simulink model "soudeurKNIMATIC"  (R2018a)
settings: Solver=VariableStepAuto  StartTime=0.0  StopTime=inf  RelTol=1e-3
StartFcn:
  | myStartFcn
model workspace: external: MATLAB File (data not in the file)
undefined symbols (not defined in the file or in its folder): deg, kg, m, mm, N, rad, s, sigbuilder_block, smiData, X, Y, Z
libraries: sm_lib x59, nesl_utility x13, robotcorelib x1, robotmaniplib x1
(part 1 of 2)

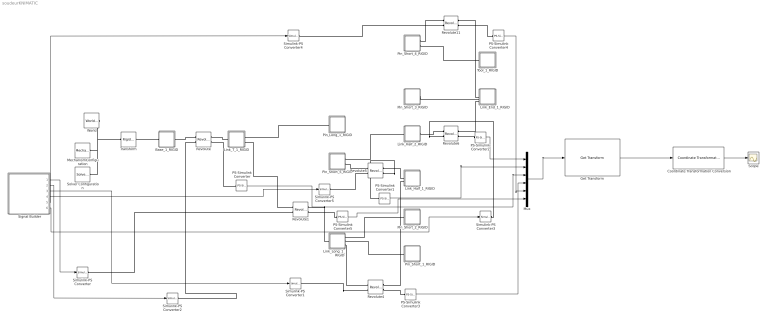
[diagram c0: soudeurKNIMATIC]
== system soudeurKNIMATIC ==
  Base_1_RIGID : Subsystem
  Coordinate Transformation Conversion : robotcorelib/Coordinate Transformation Conversion  InputRepresentation=Quaternion  InputEulerSequence=ZYX  ShowTrVecInputPort=on  OutputRepresentation=Rotation Matrix  OutputEulerSequence=ZYX  ShowTrVecOutputPort=on  SimulateUsing=Interpreted execution
  Get Transform : robotmaniplib/Get Transform  RigidBodyTree=twoJointRigidBodyTree  SourceBody=base  TargetBody=base
  Link_End_1_RIGID : Subsystem
  Link_Half_1_RIGID : Subsystem
  Link_Half_2_RIGID : Subsystem
  Link_Long_1_RIGID : Subsystem
  Link_T_1_RIGID : Subsystem
  MechanismConfiguration : sm_lib/Utilities/Mechanism Configuration  UniformGravity=Constant  GravityVector=[0 -9.80665 0]  GravityUnits=m/s^2  LinearizationDelta=0.001
  Mux : Mux  Inputs=6
  PS-Simulink Converter{,1..5} (6 alike) : nesl_utility/PS-Simulink Converter  PhysicalDomain=network_engine_domain  SubClassName=ps_output  LeftPortType=input  RightPortType=output  PseudoPeriodic=off  Frequencies=[]  Unit=1  AffineConversion=off
  Pin_Long_1_RIGID : Subsystem
  Pin_Short_1_RIGID : Subsystem
  Pin_Short_2_RIGID : Subsystem
  Pin_Short_3_RIGID : Subsystem
  Pin_Short_4_RIGID : Subsystem
  Pin_Short_5_RIGID : Subsystem
  Revolute : sm_lib/Joints/Revolute Joint  SenseConstraintForce=off  SenseConstraintForceX=off  SenseConstraintForceY=off  SenseConstraintForceZ=off  SenseConstraintTorque=off  SenseConstraintTorqueX=off  SenseConstraintTorqueY=off  SenseConstraintTorqueZ=off  SenseTotalForce=off  SenseTotalForceX=off  SenseTotalForceY=off  SenseTotalForceZ=off  SenseTotalTorque=off  SenseTotalTorqueX=off  SenseTotalTorqueY=off  SenseTotalTorqueZ=off  CompositeWrenchDir=FollowerOnBase  CompositeWrenchFrame=BaseFrame  EquilibriumPosition=0  EquilibriumPositionUnits=rad  SpringStiffness=0  SpringStiffnessUnits=N*m/rad  DampingCoefficient=0  DampingCoefficientUnits=N*m/(rad/s)  TorqueActuationMode=ComputedTorque  MotionActuationMode=InputMotion  SensePosition=on  SenseVelocity=off  SenseAcceleration=off  SenseTorqueForce=off  PositionTargetSpecify=on  PositionTargetPriority=Low  PositionTargetValue=smiData.RevoluteJoint(1).Rz.Pos  PositionTargetValueUnits=deg  VelocityTargetSpecify=off  VelocityTargetPriority=High  VelocityTargetValue=0  VelocityTargetValueUnits=deg/s
  Revolute1 : sm_lib/Joints/Revolute Joint  SenseConstraintForce=off  SenseConstraintForceX=off  SenseConstraintForceY=off  SenseConstraintForceZ=off  SenseConstraintTorque=off  SenseConstraintTorqueX=off  SenseConstraintTorqueY=off  SenseConstraintTorqueZ=off  SenseTotalForce=off  SenseTotalForceX=off  SenseTotalForceY=off  SenseTotalForceZ=off  SenseTotalTorque=off  SenseTotalTorqueX=off  SenseTotalTorqueY=off  SenseTotalTorqueZ=off  CompositeWrenchDir=FollowerOnBase  CompositeWrenchFrame=BaseFrame  EquilibriumPosition=0  EquilibriumPositionUnits=rad  SpringStiffness=0  SpringStiffnessUnits=N*m/rad  DampingCoefficient=0  DampingCoefficientUnits=N*m/(rad/s)  TorqueActuationMode=ComputedTorque  MotionActuationMode=InputMotion  SensePosition=on  SenseVelocity=off  SenseAcceleration=off  SenseTorqueForce=off  PositionTargetSpecify=on  PositionTargetPriority=Low  PositionTargetValue=smiData.RevoluteJoint(2).Rz.Pos  PositionTargetValueUnits=deg  VelocityTargetSpecify=off  VelocityTargetPriority=High  VelocityTargetValue=0  VelocityTargetValueUnits=deg/s
  Revolute11 : sm_lib/Joints/Revolute Joint  SenseConstraintForce=off  SenseConstraintForceX=off  SenseConstraintForceY=off  SenseConstraintForceZ=off  SenseConstraintTorque=off  SenseConstraintTorqueX=off  SenseConstraintTorqueY=off  SenseConstraintTorqueZ=off  SenseTotalForce=off  SenseTotalForceX=off  SenseTotalForceY=off  SenseTotalForceZ=off  SenseTotalTorque=off  SenseTotalTorqueX=off  SenseTotalTorqueY=off  SenseTotalTorqueZ=off  CompositeWrenchDir=FollowerOnBase  CompositeWrenchFrame=BaseFrame  EquilibriumPosition=0  EquilibriumPositionUnits=rad  SpringStiffness=0  SpringStiffnessUnits=N*m/rad  DampingCoefficient=0  DampingCoefficientUnits=N*m/(rad/s)  TorqueActuationMode=ComputedTorque  MotionActuationMode=InputMotion  SensePosition=on  SenseVelocity=off  SenseAcceleration=off  SenseTorqueForce=off  PositionTargetSpecify=on  PositionTargetPriority=Low  PositionTargetValue=smiData.RevoluteJoint(12).Rz.Pos  PositionTargetValueUnits=deg  VelocityTargetSpecify=off  VelocityTargetPriority=High  VelocityTargetValue=0  VelocityTargetValueUnits=deg/s
  Revolute4 : sm_lib/Joints/Revolute Joint  SenseConstraintForce=off  SenseConstraintForceX=off  SenseConstraintForceY=off  SenseConstraintForceZ=off  SenseConstraintTorque=off  SenseConstraintTorqueX=off  SenseConstraintTorqueY=off  SenseConstraintTorqueZ=off  SenseTotalForce=off  SenseTotalForceX=off  SenseTotalForceY=off  SenseTotalForceZ=off  SenseTotalTorque=off  SenseTotalTorqueX=off  SenseTotalTorqueY=off  SenseTotalTorqueZ=off  CompositeWrenchDir=FollowerOnBase  CompositeWrenchFrame=BaseFrame  EquilibriumPosition=0  EquilibriumPositionUnits=rad  SpringStiffness=0  SpringStiffnessUnits=N*m/rad  DampingCoefficient=0  DampingCoefficientUnits=N*m/(rad/s)  TorqueActuationMode=ComputedTorque  MotionActuationMode=InputMotion  SensePosition=on  SenseVelocity=off  SenseAcceleration=off  SenseTorqueForce=off  PositionTargetSpecify=on  PositionTargetPriority=Low  PositionTargetValue=smiData.RevoluteJoint(5).Rz.Pos  PositionTargetValueUnits=deg  VelocityTargetSpecify=off  VelocityTargetPriority=High  VelocityTargetValue=0  VelocityTargetValueUnits=deg/s
  Revolute5 : sm_lib/Joints/Revolute Joint  SenseConstraintForce=off  SenseConstraintForceX=off  SenseConstraintForceY=off  SenseConstraintForceZ=off  SenseConstraintTorque=off  SenseConstraintTorqueX=off  SenseConstraintTorqueY=off  SenseConstraintTorqueZ=off  SenseTotalForce=off  SenseTotalForceX=off  SenseTotalForceY=off  SenseTotalForceZ=off  SenseTotalTorque=off  SenseTotalTorqueX=off  SenseTotalTorqueY=off  SenseTotalTorqueZ=off  CompositeWrenchDir=FollowerOnBase  CompositeWrenchFrame=BaseFrame  EquilibriumPosition=0  EquilibriumPositionUnits=rad  SpringStiffness=0  SpringStiffnessUnits=N*m/rad  DampingCoefficient=0  DampingCoefficientUnits=N*m/(rad/s)  TorqueActuationMode=ComputedTorque  MotionActuationMode=InputMotion  SensePosition=on  SenseVelocity=off  SenseAcceleration=off  SenseTorqueForce=off  PositionTargetSpecify=on  PositionTargetPriority=Low  PositionTargetValue=smiData.RevoluteJoint(6).Rz.Pos  PositionTargetValueUnits=deg  VelocityTargetSpecify=off  VelocityTargetPriority=High  VelocityTargetValue=0  VelocityTargetValueUnits=deg/s
  Revolute6 : sm_lib/Joints/Revolute Joint  SenseConstraintForce=off  SenseConstraintForceX=off  SenseConstraintForceY=off  SenseConstraintForceZ=off  SenseConstraintTorque=off  SenseConstraintTorqueX=off  SenseConstraintTorqueY=off  SenseConstraintTorqueZ=off  SenseTotalForce=off  SenseTotalForceX=off  SenseTotalForceY=off  SenseTotalForceZ=off  SenseTotalTorque=off  SenseTotalTorqueX=off  SenseTotalTorqueY=off  SenseTotalTorqueZ=off  CompositeWrenchDir=FollowerOnBase  CompositeWrenchFrame=BaseFrame  EquilibriumPosition=0  EquilibriumPositionUnits=rad  SpringStiffness=0  SpringStiffnessUnits=N*m/rad  DampingCoefficient=0  DampingCoefficientUnits=N*m/(rad/s)  TorqueActuationMode=ComputedTorque  MotionActuationMode=InputMotion  SensePosition=on  SenseVelocity=off  SenseAcceleration=off  SenseTorqueForce=off  PositionTargetSpecify=on  PositionTargetPriority=Low  PositionTargetValue=smiData.RevoluteJoint(7).Rz.Pos  PositionTargetValueUnits=deg  VelocityTargetSpecify=off  VelocityTargetPriority=High  VelocityTargetValue=0  VelocityTargetValueUnits=deg/s
  Scope : Scope
  Signal Builder : Subsystem  Tag=STV Subsys  LoadFcn=sigbuilder_block('load');  StartFcn=sigbuilder_block('start');  StopFcn=sigbuilder_block('stop');  ClipboardFcn=sigbuilder_block('clipboard');  mask(Sigbuilder block){tuvar=[0:10]}
      mask help: Simulink:masks:SigbuilderBlock_MD
      mask init:
      | if ~strcmp(get_param(bdroot(gcbh),'SimulationStatus'),'stopped') tuvar = sigbuilder_block('maskInit'); end
  Simulink-PS Converter{,1..4} (5 alike) : nesl_utility/Simulink-PS Converter  PhysicalDomain=network_engine_domain  SubClassName=ps_input  LeftPortType=input  RightPortType=output  PseudoPeriodic=off  Frequencies=[]  NoiseDistribution=none  NoiseParameters=[]  Unit=rad  AffineConversion=off  FilteringAndDerivatives=filter  SimscapeFilterOrder=2  InputFilterTimeConstant=0.001  UdotUserProvided=0
  Simulink-PS Converter5 : nesl_utility/Simulink-PS Converter  PhysicalDomain=network_engine_domain  SubClassName=ps_input  LeftPortType=input  RightPortType=output  PseudoPeriodic=off  Frequencies=[]  NoiseDistribution=none  NoiseParameters=[]  Unit=1  AffineConversion=off  FilteringAndDerivatives=provide  SimscapeFilterOrder=1  InputFilterTimeConstant=0.001  UdotUserProvided=0
  Solver Configuration : nesl_utility/Solver Configuration  PhysicalDomain=network_engine_domain  SubClassName=solver  LeftPortType=input  RightPortType=generic  Tones=[]  Harmonics=[]  SimulateNoise=off  Profile=off  UseLocalSampling=off  EnableSwitchedLinearOptims=on  FrequencyDomain=off  UseCCode=off  RelTol=0.001  AbsTol=1e-06  MinStep=1e-09  ToWorkspace=off  RevertToSquareIcSolve=off  NumHomotopyIterations=100  PhasorMode=off  PhasorModeNumHarmonics=1  DoDC=off  ResidualTolerance=1e-09  UseLocalSolver=off  LocalSolverChoice=NE_BACKWARD_EULER_ADVANCER  LocalSolverSampleTime=0.001  DoFixedCost=off  MaxNonlinIter=3  MaxModeIter=2  LinearAlgebra=Sparse  EquationFormulation=NE_TIME_EF  DelaysMemoryBudget=1024  AutomaticFiltering=on  FilteringTimeConstant=0.001
  Tool_1_RIGID : Subsystem
  Transform : sm_lib/Frames and Transforms/Rigid Transform  TranslationMethod=Cartesian  TranslationStandardOffset=0  TranslationLengthUnit=mm  TranslationStandardAxis=+Z  TranslationCartesianOffset=smiData.RigidTransform(25).translation  TranslationROffset=0  TranslationROffsetUnits=m  TranslationZOffset=0  TranslationZOffsetUnits=m  TranslationThetaOffset=0  TranslationThetaOffsetUnits=deg  RotationMethod=ArbitraryAxis  RotationAngleUnits=rad  RotationStandardAxis=+Z  RotationAngle=smiData.RigidTransform(25).angle  RotationArbitraryAxis=smiData.RigidTransform(25).axis  FollAlignAxisA=+X  BaseAlignAxisA=+Y  FollAlignAxisB=+Y  BaseAlignAxisB=+Z  RotationSequenceAxes=FollowerAxes  RotationSequence=XYX  RotationSequenceAngles=[0 0 0]  RotationSequenceAnglesUnits=deg  RotationMatrix=[1 0 0; 0 1 0; 0 0 1]
  World : sm_lib/Frames and Transforms/World Frame
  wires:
  Signal Builder/1(Signal 1) -> Simulink-PS Converter/1
  Signal Builder/2(Signal 2) -> Simulink-PS Converter2/1
  Signal Builder/3(Signal 3) -> Simulink-PS Converter1/1
  Signal Builder/4(Signal 4) -> Simulink-PS Converter5/1
  Signal Builder/5(Signal 5) -> Simulink-PS Converter4/1
  Signal Builder/6(Signal 6) -> Simulink-PS Converter3/1
  Get Transform/1 -> Coordinate Transformation Conversion/1
  PS-Simulink Converter2/1 -> Mux/1
  PS-Simulink Converter1/1 -> Mux/2
  PS-Simulink Converter/1 -> Mux/3
  PS-Simulink Converter3/1 -> Mux/4
  PS-Simulink Converter4/1 -> Mux/5
  PS-Simulink Converter5/1 -> Mux/6
  Mux/1 -> Get Transform/1
  Coordinate Transformation Conversion/1 -> Scope/1
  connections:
  MechanismConfiguration/RConn1 -- Transform/LConn1 -- World/RConn1 -- Solver Configuration/RConn1
  Base_1_RIGID/RConn1 -- Revolute/LConn1
  Link_Half_1_RIGID/LConn2 -- Revolute4/RConn1
  Pin_Short_5_RIGID/RConn2 -- Revolute5/LConn1
  Link_Half_1_RIGID/LConn1 -- Revolute5/RConn1
  Link_Half_2_RIGID/RConn1 -- Revolute6/LConn1
  Link_End_1_RIGID/LConn3 -- Revolute6/RConn1
  Pin_Short_5_RIGID/RConn1 -- Link_Half_2_RIGID/LConn1
  Link_Long_1_RIGID/RConn2 -- Pin_Short_1_RIGID/LConn1
  Link_T_1_RIGID/LConn1 -- Revolute/RConn1
  Link_Long_1_RIGID/RConn1 -- Pin_Short_2_RIGID/LConn1
  Pin_Short_3_RIGID/RConn1 -- Link_End_1_RIGID/LConn2
  Pin_Short_4_RIGID/RConn1 -- Revolute11/LConn1
  Link_End_1_RIGID/LConn1 -- Revolute11/RConn1
  Base_1_RIGID/LConn1 -- Transform/RConn1
  Link_T_1_RIGID/RConn2 -- Revolute1/LConn1
  Link_Long_1_RIGID/LConn1 -- Revolute1/RConn1
  Link_T_1_RIGID/RConn1 -- Pin_Long_1_RIGID/LConn1
  Pin_Short_4_RIGID/RConn2 -- Tool_1_RIGID/LConn1
  Link_Long_1_RIGID/RConn3 -- Revolute4/LConn1
  Simulink-PS Converter/RConn1 -- Revolute1/LConn2
  Simulink-PS Converter2/RConn1 -- Revolute/LConn2
  Simulink-PS Converter5/RConn1 -- Revolute5/LConn2
  Simulink-PS Converter1/RConn1 -- Revolute4/LConn2
  Simulink-PS Converter3/RConn1 -- Revolute6/LConn2
  Simulink-PS Converter4/RConn1 -- Revolute11/LConn2
  PS-Simulink Converter/LConn1 -- Revolute/RConn2
  PS-Simulink Converter1/LConn1 -- Revolute5/RConn2
  PS-Simulink Converter2/LConn1 -- Revolute6/RConn2
  PS-Simulink Converter3/LConn1 -- Revolute4/RConn2
  PS-Simulink Converter4/LConn1 -- Revolute11/RConn2
  PS-Simulink Converter5/LConn1 -- Revolute1/RConn2

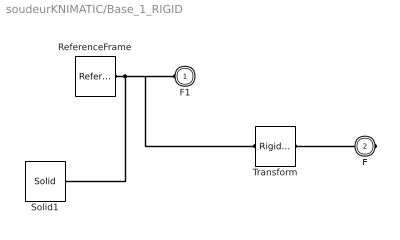
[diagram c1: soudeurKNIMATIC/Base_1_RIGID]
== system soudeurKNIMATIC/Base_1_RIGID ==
  ReferenceFrame : sm_lib/Frames and Transforms/Reference Frame
  Solid1 : sm_lib/Body Elements/Solid  InertiaType=Custom  Mass=smiData.Solid(4).mass  MassUnits=kg  CenterOfMass=smiData.Solid(4).CoM  CenterOfMassUnits=mm  MomentsOfInertia=smiData.Solid(4).MoI  MomentsOfInertiaUnits=kg*mm^2  ProductsOfInertia=smiData.Solid(4).PoI  ProductsOfInertiaUnits=kg*mm^2  DensityBased=on  Density=1000  DensityUnits=kg/m^3  DoExposeReferenceFrame=on  SerializedFrames=<Frames/>  GraphicType=FromGeometry  MarkerShape=Sphere  MarkerSize=10  GraphicVisPropType=SimpleVisualProperties  GraphicDiffuseColor=smiData.Solid(4).color  GraphicSpecularColor=[0.5 0.5 0.5 1.0]  GraphicAmbientColor=[0.15 0.15 0.15 1.0]  GraphicEmissiveColor=[0.0 0.0 0.0 1.0]  GraphicShininess=75  GraphicOpacity=smiData.Solid(4).opacity  GeometryShape=FromFile  RectangleSize=[1 1]  RectangleSizeUnits=m  BrickDimensions=[1 1 1]  BrickDimensionUnits=m  CylinderRadius=1  CylinderRadiusUnits=m  CylinderLength=1  CylinderLengthUnits=m  SphereRadius=1  SphereRadiusUnits=m  EllipsoidRadii=[1 1 1]  EllipsoidRadiiUnits=m  ExtrusionCrossSection=[1 1; -1 1; -1 -1; 1 -1]  ExtrusionCrossSectionUnits=m  ExtrusionLength=1  ExtrusionLengthUnits=m  PolygonNumSides=3  PolygonOuterRadius=1  PolygonOuterRadiusUnits=m  ExtGeomFileType=STEP  ExtGeomFileName=Link_End_Default_sldprt.STEP  ExtGeomFileUnits=m  RevolutionCrossSection=[1 1; 1 -1; 2 -1; 2 1]  RevolutionCrossSectionUnits=m  RevolutionExtent=Full  RevolutionAngle=180  RevolutionAngleUnits=deg
  Transform : sm_lib/Frames and Transforms/Rigid Transform  TranslationMethod=Cartesian  TranslationStandardOffset=0  TranslationLengthUnit=mm  TranslationStandardAxis=+Z  TranslationCartesianOffset=smiData.RigidTransform(1).translation  TranslationROffset=0  TranslationROffsetUnits=m  TranslationZOffset=0  TranslationZOffsetUnits=m  TranslationThetaOffset=0  TranslationThetaOffsetUnits=deg  RotationMethod=ArbitraryAxis  RotationAngleUnits=rad  RotationStandardAxis=+Z  RotationAngle=smiData.RigidTransform(1).angle  RotationArbitraryAxis=smiData.RigidTransform(1).axis  FollAlignAxisA=+X  BaseAlignAxisA=+Y  FollAlignAxisB=+Y  BaseAlignAxisB=+Z  RotationSequenceAxes=FollowerAxes  RotationSequence=XYX  RotationSequenceAngles=[0 0 0]  RotationSequenceAnglesUnits=deg  RotationMatrix=[1 0 0; 0 1 0; 0 0 1]
  F1 : PMIOPort  Side=Left
  F : PMIOPort  Port=2  Side=Right
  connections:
  ReferenceFrame/RConn1 -- Solid1/RConn1 -- Transform/LConn1 -- F1/RConn1
  Transform/RConn1 -- F/RConn1

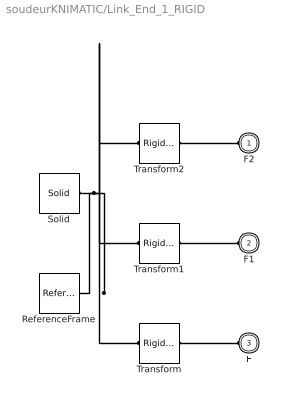
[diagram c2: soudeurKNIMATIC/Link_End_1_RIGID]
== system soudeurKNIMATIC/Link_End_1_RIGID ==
  ReferenceFrame : sm_lib/Frames and Transforms/Reference Frame
  Solid : sm_lib/Body Elements/Solid  InertiaType=Custom  Mass=smiData.Solid(4).mass  MassUnits=kg  CenterOfMass=smiData.Solid(4).CoM  CenterOfMassUnits=mm  MomentsOfInertia=smiData.Solid(4).MoI  MomentsOfInertiaUnits=kg*mm^2  ProductsOfInertia=smiData.Solid(4).PoI  ProductsOfInertiaUnits=kg*mm^2  DensityBased=on  Density=1000  DensityUnits=kg/m^3  DoExposeReferenceFrame=on  SerializedFrames=<Frames/>  GraphicType=FromGeometry  MarkerShape=Sphere  MarkerSize=10  GraphicVisPropType=SimpleVisualProperties  GraphicDiffuseColor=smiData.Solid(4).color  GraphicSpecularColor=[0.5 0.5 0.5 1.0]  GraphicAmbientColor=[0.15 0.15 0.15 1.0]  GraphicEmissiveColor=[0.0 0.0 0.0 1.0]  GraphicShininess=75  GraphicOpacity=smiData.Solid(4).opacity  GeometryShape=FromFile  RectangleSize=[1 1]  RectangleSizeUnits=m  BrickDimensions=[1 1 1]  BrickDimensionUnits=m  CylinderRadius=1  CylinderRadiusUnits=m  CylinderLength=1  CylinderLengthUnits=m  SphereRadius=1  SphereRadiusUnits=m  EllipsoidRadii=[1 1 1]  EllipsoidRadiiUnits=m  ExtrusionCrossSection=[1 1; -1 1; -1 -1; 1 -1]  ExtrusionCrossSectionUnits=m  ExtrusionLength=1  ExtrusionLengthUnits=m  PolygonNumSides=3  PolygonOuterRadius=1  PolygonOuterRadiusUnits=m  ExtGeomFileType=STEP  ExtGeomFileName=Link_End_Default_sldprt.STEP  ExtGeomFileUnits=m  RevolutionCrossSection=[1 1; 1 -1; 2 -1; 2 1]  RevolutionCrossSectionUnits=m  RevolutionExtent=Full  RevolutionAngle=180  RevolutionAngleUnits=deg
  Transform : sm_lib/Frames and Transforms/Rigid Transform  TranslationMethod=Cartesian  TranslationStandardOffset=0  TranslationLengthUnit=mm  TranslationStandardAxis=+Z  TranslationCartesianOffset=smiData.RigidTransform(14).translation  TranslationROffset=0  TranslationROffsetUnits=m  TranslationZOffset=0  TranslationZOffsetUnits=m  TranslationThetaOffset=0  TranslationThetaOffsetUnits=deg  RotationMethod=ArbitraryAxis  RotationAngleUnits=rad  RotationStandardAxis=+Z  RotationAngle=smiData.RigidTransform(14).angle  RotationArbitraryAxis=smiData.RigidTransform(14).axis  FollAlignAxisA=+X  BaseAlignAxisA=+Y  FollAlignAxisB=+Y  BaseAlignAxisB=+Z  RotationSequenceAxes=FollowerAxes  RotationSequence=XYX  RotationSequenceAngles=[0 0 0]  RotationSequenceAnglesUnits=deg  RotationMatrix=[1 0 0; 0 1 0; 0 0 1]
  Transform1 : sm_lib/Frames and Transforms/Rigid Transform  TranslationMethod=Cartesian  TranslationStandardOffset=0  TranslationLengthUnit=mm  TranslationStandardAxis=+Z  TranslationCartesianOffset=smiData.RigidTransform(22).translation  TranslationROffset=0  TranslationROffsetUnits=m  TranslationZOffset=0  TranslationZOffsetUnits=m  TranslationThetaOffset=0  TranslationThetaOffsetUnits=deg  RotationMethod=ArbitraryAxis  RotationAngleUnits=rad  RotationStandardAxis=+Z  RotationAngle=smiData.RigidTransform(22).angle  RotationArbitraryAxis=smiData.RigidTransform(22).axis  FollAlignAxisA=+X  BaseAlignAxisA=+Y  FollAlignAxisB=+Y  BaseAlignAxisB=+Z  RotationSequenceAxes=FollowerAxes  RotationSequence=XYX  RotationSequenceAngles=[0 0 0]  RotationSequenceAnglesUnits=deg  RotationMatrix=[1 0 0; 0 1 0; 0 0 1]
  Transform2 : sm_lib/Frames and Transforms/Rigid Transform  TranslationMethod=Cartesian  TranslationStandardOffset=0  TranslationLengthUnit=mm  TranslationStandardAxis=+Z  TranslationCartesianOffset=smiData.RigidTransform(24).translation  TranslationROffset=0  TranslationROffsetUnits=m  TranslationZOffset=0  TranslationZOffsetUnits=m  TranslationThetaOffset=0  TranslationThetaOffsetUnits=deg  RotationMethod=ArbitraryAxis  RotationAngleUnits=rad  RotationStandardAxis=+Z  RotationAngle=smiData.RigidTransform(24).angle  RotationArbitraryAxis=smiData.RigidTransform(24).axis  FollAlignAxisA=+X  BaseAlignAxisA=+Y  FollAlignAxisB=+Y  BaseAlignAxisB=+Z  RotationSequenceAxes=FollowerAxes  RotationSequence=XYX  RotationSequenceAngles=[0 0 0]  RotationSequenceAnglesUnits=deg  RotationMatrix=[1 0 0; 0 1 0; 0 0 1]
  F2 : PMIOPort  Side=Left
  F1 : PMIOPort  Port=2  Side=Left
  F : PMIOPort  Port=3  Side=Left
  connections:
  Solid/RConn1 -- ReferenceFrame/RConn1 -- Transform1/LConn1 -- Transform2/LConn1 -- Transform/LConn1
  Transform/RConn1 -- F/RConn1
  Transform1/RConn1 -- F1/RConn1
  Transform2/RConn1 -- F2/RConn1

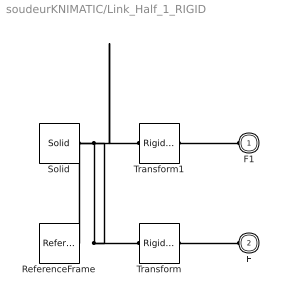
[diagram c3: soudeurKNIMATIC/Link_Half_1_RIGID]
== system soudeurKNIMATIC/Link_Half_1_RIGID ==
  ReferenceFrame : sm_lib/Frames and Transforms/Reference Frame
  Solid : sm_lib/Body Elements/Solid  InertiaType=Custom  Mass=smiData.Solid(6).mass  MassUnits=kg  CenterOfMass=smiData.Solid(6).CoM  CenterOfMassUnits=mm  MomentsOfInertia=smiData.Solid(6).MoI  MomentsOfInertiaUnits=kg*mm^2  ProductsOfInertia=smiData.Solid(6).PoI  ProductsOfInertiaUnits=kg*mm^2  DensityBased=on  Density=1000  DensityUnits=kg/m^3  DoExposeReferenceFrame=on  SerializedFrames=<Frames/>  GraphicType=FromGeometry  MarkerShape=Sphere  MarkerSize=10  GraphicVisPropType=SimpleVisualProperties  GraphicDiffuseColor=smiData.Solid(6).color  GraphicSpecularColor=[0.5 0.5 0.5 1.0]  GraphicAmbientColor=[0.15 0.15 0.15 1.0]  GraphicEmissiveColor=[0.0 0.0 0.0 1.0]  GraphicShininess=75  GraphicOpacity=smiData.Solid(6).opacity  GeometryShape=FromFile  RectangleSize=[1 1]  RectangleSizeUnits=m  BrickDimensions=[1 1 1]  BrickDimensionUnits=m  CylinderRadius=1  CylinderRadiusUnits=m  CylinderLength=1  CylinderLengthUnits=m  SphereRadius=1  SphereRadiusUnits=m  EllipsoidRadii=[1 1 1]  EllipsoidRadiiUnits=m  ExtrusionCrossSection=[1 1; -1 1; -1 -1; 1 -1]  ExtrusionCrossSectionUnits=m  ExtrusionLength=1  ExtrusionLengthUnits=m  PolygonNumSides=3  PolygonOuterRadius=1  PolygonOuterRadiusUnits=m  ExtGeomFileType=STEP  ExtGeomFileName=Link_Half_Default_sldprt.STEP  ExtGeomFileUnits=m  RevolutionCrossSection=[1 1; 1 -1; 2 -1; 2 1]  RevolutionCrossSectionUnits=m  RevolutionExtent=Full  RevolutionAngle=180  RevolutionAngleUnits=deg
  Transform : sm_lib/Frames and Transforms/Rigid Transform  TranslationMethod=Cartesian  TranslationStandardOffset=0  TranslationLengthUnit=mm  TranslationStandardAxis=+Z  TranslationCartesianOffset=smiData.RigidTransform(10).translation  TranslationROffset=0  TranslationROffsetUnits=m  TranslationZOffset=0  TranslationZOffsetUnits=m  TranslationThetaOffset=0  TranslationThetaOffsetUnits=deg  RotationMethod=ArbitraryAxis  RotationAngleUnits=rad  RotationStandardAxis=+Z  RotationAngle=smiData.RigidTransform(10).angle  RotationArbitraryAxis=smiData.RigidTransform(10).axis  FollAlignAxisA=+X  BaseAlignAxisA=+Y  FollAlignAxisB=+Y  BaseAlignAxisB=+Z  RotationSequenceAxes=FollowerAxes  RotationSequence=XYX  RotationSequenceAngles=[0 0 0]  RotationSequenceAnglesUnits=deg  RotationMatrix=[1 0 0; 0 1 0; 0 0 1]
  Transform1 : sm_lib/Frames and Transforms/Rigid Transform  TranslationMethod=Cartesian  TranslationStandardOffset=0  TranslationLengthUnit=mm  TranslationStandardAxis=+Z  TranslationCartesianOffset=smiData.RigidTransform(12).translation  TranslationROffset=0  TranslationROffsetUnits=m  TranslationZOffset=0  TranslationZOffsetUnits=m  TranslationThetaOffset=0  TranslationThetaOffsetUnits=deg  RotationMethod=ArbitraryAxis  RotationAngleUnits=rad  RotationStandardAxis=+Z  RotationAngle=smiData.RigidTransform(12).angle  RotationArbitraryAxis=smiData.RigidTransform(12).axis  FollAlignAxisA=+X  BaseAlignAxisA=+Y  FollAlignAxisB=+Y  BaseAlignAxisB=+Z  RotationSequenceAxes=FollowerAxes  RotationSequence=XYX  RotationSequenceAngles=[0 0 0]  RotationSequenceAnglesUnits=deg  RotationMatrix=[1 0 0; 0 1 0; 0 0 1]
  F1 : PMIOPort  Side=Left
  F : PMIOPort  Port=2  Side=Left
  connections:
  Solid/RConn1 -- ReferenceFrame/RConn1 -- Transform/LConn1 -- Transform1/LConn1
  Transform/RConn1 -- F/RConn1
  Transform1/RConn1 -- F1/RConn1

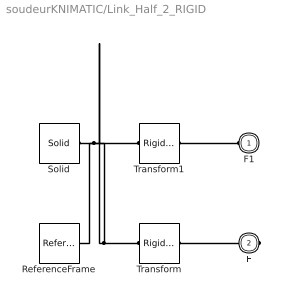
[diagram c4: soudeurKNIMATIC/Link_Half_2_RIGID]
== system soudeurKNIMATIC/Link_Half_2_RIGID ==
  ReferenceFrame : sm_lib/Frames and Transforms/Reference Frame
  Solid : sm_lib/Body Elements/Solid  InertiaType=Custom  Mass=smiData.Solid(6).mass  MassUnits=kg  CenterOfMass=smiData.Solid(6).CoM  CenterOfMassUnits=mm  MomentsOfInertia=smiData.Solid(6).MoI  MomentsOfInertiaUnits=kg*mm^2  ProductsOfInertia=smiData.Solid(6).PoI  ProductsOfInertiaUnits=kg*mm^2  DensityBased=on  Density=1000  DensityUnits=kg/m^3  DoExposeReferenceFrame=on  SerializedFrames=<Frames/>  GraphicType=FromGeometry  MarkerShape=Sphere  MarkerSize=10  GraphicVisPropType=SimpleVisualProperties  GraphicDiffuseColor=smiData.Solid(6).color  GraphicSpecularColor=[0.5 0.5 0.5 1.0]  GraphicAmbientColor=[0.15 0.15 0.15 1.0]  GraphicEmissiveColor=[0.0 0.0 0.0 1.0]  GraphicShininess=75  GraphicOpacity=smiData.Solid(6).opacity  GeometryShape=FromFile  RectangleSize=[1 1]  RectangleSizeUnits=m  BrickDimensions=[1 1 1]  BrickDimensionUnits=m  CylinderRadius=1  CylinderRadiusUnits=m  CylinderLength=1  CylinderLengthUnits=m  SphereRadius=1  SphereRadiusUnits=m  EllipsoidRadii=[1 1 1]  EllipsoidRadiiUnits=m  ExtrusionCrossSection=[1 1; -1 1; -1 -1; 1 -1]  ExtrusionCrossSectionUnits=m  ExtrusionLength=1  ExtrusionLengthUnits=m  PolygonNumSides=3  PolygonOuterRadius=1  PolygonOuterRadiusUnits=m  ExtGeomFileType=STEP  ExtGeomFileName=Link_Half_Default_sldprt.STEP  ExtGeomFileUnits=m  RevolutionCrossSection=[1 1; 1 -1; 2 -1; 2 1]  RevolutionCrossSectionUnits=m  RevolutionExtent=Full  RevolutionAngle=180  RevolutionAngleUnits=deg
  Transform : sm_lib/Frames and Transforms/Rigid Transform  TranslationMethod=Cartesian  TranslationStandardOffset=0  TranslationLengthUnit=mm  TranslationStandardAxis=+Z  TranslationCartesianOffset=smiData.RigidTransform(13).translation  TranslationROffset=0  TranslationROffsetUnits=m  TranslationZOffset=0  TranslationZOffsetUnits=m  TranslationThetaOffset=0  TranslationThetaOffsetUnits=deg  RotationMethod=ArbitraryAxis  RotationAngleUnits=rad  RotationStandardAxis=+Z  RotationAngle=smiData.RigidTransform(13).angle  RotationArbitraryAxis=smiData.RigidTransform(13).axis  FollAlignAxisA=+X  BaseAlignAxisA=+Y  FollAlignAxisB=+Y  BaseAlignAxisB=+Z  RotationSequenceAxes=FollowerAxes  RotationSequence=XYX  RotationSequenceAngles=[0 0 0]  RotationSequenceAnglesUnits=deg  RotationMatrix=[1 0 0; 0 1 0; 0 0 1]
  Transform1 : sm_lib/Frames and Transforms/Rigid Transform  TranslationMethod=Cartesian  TranslationStandardOffset=0  TranslationLengthUnit=mm  TranslationStandardAxis=+Z  TranslationCartesianOffset=smiData.RigidTransform(16).translation  TranslationROffset=0  TranslationROffsetUnits=m  TranslationZOffset=0  TranslationZOffsetUnits=m  TranslationThetaOffset=0  TranslationThetaOffsetUnits=deg  RotationMethod=ArbitraryAxis  RotationAngleUnits=rad  RotationStandardAxis=+Z  RotationAngle=smiData.RigidTransform(16).angle  RotationArbitraryAxis=smiData.RigidTransform(16).axis  FollAlignAxisA=+X  BaseAlignAxisA=+Y  FollAlignAxisB=+Y  BaseAlignAxisB=+Z  RotationSequenceAxes=FollowerAxes  RotationSequence=XYX  RotationSequenceAngles=[0 0 0]  RotationSequenceAnglesUnits=deg  RotationMatrix=[1 0 0; 0 1 0; 0 0 1]
  F1 : PMIOPort  Side=Left
  F : PMIOPort  Port=2  Side=Right
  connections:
  Solid/RConn1 -- ReferenceFrame/RConn1 -- Transform/LConn1 -- Transform1/LConn1
  Transform/RConn1 -- F/RConn1
  Transform1/RConn1 -- F1/RConn1

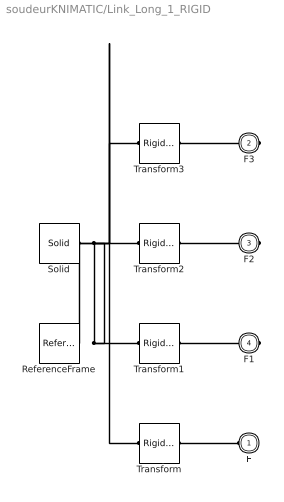
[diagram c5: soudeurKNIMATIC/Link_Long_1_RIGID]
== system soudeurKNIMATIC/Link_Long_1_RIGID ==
  ReferenceFrame : sm_lib/Frames and Transforms/Reference Frame
  Solid : sm_lib/Body Elements/Solid  InertiaType=Custom  Mass=smiData.Solid(8).mass  MassUnits=kg  CenterOfMass=smiData.Solid(8).CoM  CenterOfMassUnits=mm  MomentsOfInertia=smiData.Solid(8).MoI  MomentsOfInertiaUnits=kg*mm^2  ProductsOfInertia=smiData.Solid(8).PoI  ProductsOfInertiaUnits=kg*mm^2  DensityBased=on  Density=1000  DensityUnits=kg/m^3  DoExposeReferenceFrame=on  SerializedFrames=<Frames/>  GraphicType=FromGeometry  MarkerShape=Sphere  MarkerSize=10  GraphicVisPropType=SimpleVisualProperties  GraphicDiffuseColor=smiData.Solid(8).color  GraphicSpecularColor=[0.5 0.5 0.5 1.0]  GraphicAmbientColor=[0.15 0.15 0.15 1.0]  GraphicEmissiveColor=[0.0 0.0 0.0 1.0]  GraphicShininess=75  GraphicOpacity=smiData.Solid(8).opacity  GeometryShape=FromFile  RectangleSize=[1 1]  RectangleSizeUnits=m  BrickDimensions=[1 1 1]  BrickDimensionUnits=m  CylinderRadius=1  CylinderRadiusUnits=m  CylinderLength=1  CylinderLengthUnits=m  SphereRadius=1  SphereRadiusUnits=m  EllipsoidRadii=[1 1 1]  EllipsoidRadiiUnits=m  ExtrusionCrossSection=[1 1; -1 1; -1 -1; 1 -1]  ExtrusionCrossSectionUnits=m  ExtrusionLength=1  ExtrusionLengthUnits=m  PolygonNumSides=3  PolygonOuterRadius=1  PolygonOuterRadiusUnits=m  ExtGeomFileType=STEP  ExtGeomFileName=Link_Long_Default_sldprt.STEP  ExtGeomFileUnits=m  RevolutionCrossSection=[1 1; 1 -1; 2 -1; 2 1]  RevolutionCrossSectionUnits=m  RevolutionExtent=Full  RevolutionAngle=180  RevolutionAngleUnits=deg
  Transform : sm_lib/Frames and Transforms/Rigid Transform  TranslationMethod=Cartesian  TranslationStandardOffset=0  TranslationLengthUnit=mm  TranslationStandardAxis=+Z  TranslationCartesianOffset=smiData.RigidTransform(4).translation  TranslationROffset=0  TranslationROffsetUnits=m  TranslationZOffset=0  TranslationZOffsetUnits=m  TranslationThetaOffset=0  TranslationThetaOffsetUnits=deg  RotationMethod=ArbitraryAxis  RotationAngleUnits=rad  RotationStandardAxis=+Z  RotationAngle=smiData.RigidTransform(4).angle  RotationArbitraryAxis=smiData.RigidTransform(4).axis  FollAlignAxisA=+X  BaseAlignAxisA=+Y  FollAlignAxisB=+Y  BaseAlignAxisB=+Z  RotationSequenceAxes=FollowerAxes  RotationSequence=XYX  RotationSequenceAngles=[0 0 0]  RotationSequenceAnglesUnits=deg  RotationMatrix=[1 0 0; 0 1 0; 0 0 1]
  Transform1 : sm_lib/Frames and Transforms/Rigid Transform  TranslationMethod=Cartesian  TranslationStandardOffset=0  TranslationLengthUnit=mm  TranslationStandardAxis=+Z  TranslationCartesianOffset=smiData.RigidTransform(9).translation  TranslationROffset=0  TranslationROffsetUnits=m  TranslationZOffset=0  TranslationZOffsetUnits=m  TranslationThetaOffset=0  TranslationThetaOffsetUnits=deg  RotationMethod=ArbitraryAxis  RotationAngleUnits=rad  RotationStandardAxis=+Z  RotationAngle=smiData.RigidTransform(9).angle  RotationArbitraryAxis=smiData.RigidTransform(9).axis  FollAlignAxisA=+X  BaseAlignAxisA=+Y  FollAlignAxisB=+Y  BaseAlignAxisB=+Z  RotationSequenceAxes=FollowerAxes  RotationSequence=XYX  RotationSequenceAngles=[0 0 0]  RotationSequenceAnglesUnits=deg  RotationMatrix=[1 0 0; 0 1 0; 0 0 1]
  Transform2 : sm_lib/Frames and Transforms/Rigid Transform  TranslationMethod=Cartesian  TranslationStandardOffset=0  TranslationLengthUnit=mm  TranslationStandardAxis=+Z  TranslationCartesianOffset=smiData.RigidTransform(17).translation  TranslationROffset=0  TranslationROffsetUnits=m  TranslationZOffset=0  TranslationZOffsetUnits=m  TranslationThetaOffset=0  TranslationThetaOffsetUnits=deg  RotationMethod=ArbitraryAxis  RotationAngleUnits=rad  RotationStandardAxis=+Z  RotationAngle=smiData.RigidTransform(17).angle  RotationArbitraryAxis=smiData.RigidTransform(17).axis  FollAlignAxisA=+X  BaseAlignAxisA=+Y  FollAlignAxisB=+Y  BaseAlignAxisB=+Z  RotationSequenceAxes=FollowerAxes  RotationSequence=XYX  RotationSequenceAngles=[0 0 0]  RotationSequenceAnglesUnits=deg  RotationMatrix=[1 0 0; 0 1 0; 0 0 1]
  Transform3 : sm_lib/Frames and Transforms/Rigid Transform  TranslationMethod=Cartesian  TranslationStandardOffset=0  TranslationLengthUnit=mm  TranslationStandardAxis=+Z  TranslationCartesianOffset=smiData.RigidTransform(19).translation  TranslationROffset=0  TranslationROffsetUnits=m  TranslationZOffset=0  TranslationZOffsetUnits=m  TranslationThetaOffset=0  TranslationThetaOffsetUnits=deg  RotationMethod=ArbitraryAxis  RotationAngleUnits=rad  RotationStandardAxis=+Z  RotationAngle=smiData.RigidTransform(19).angle  RotationArbitraryAxis=smiData.RigidTransform(19).axis  FollAlignAxisA=+X  BaseAlignAxisA=+Y  FollAlignAxisB=+Y  BaseAlignAxisB=+Z  RotationSequenceAxes=FollowerAxes  RotationSequence=XYX  RotationSequenceAngles=[0 0 0]  RotationSequenceAnglesUnits=deg  RotationMatrix=[1 0 0; 0 1 0; 0 0 1]
  F : PMIOPort  Side=Left
  F3 : PMIOPort  Port=2  Side=Right
  F2 : PMIOPort  Port=3  Side=Right
  F1 : PMIOPort  Port=4  Side=Right
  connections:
  Solid/RConn1 -- ReferenceFrame/RConn1 -- Transform/LConn1 -- Transform1/LConn1 -- Transform2/LConn1 -- Transform3/LConn1
  Transform/RConn1 -- F/RConn1
  Transform1/RConn1 -- F1/RConn1
  Transform2/RConn1 -- F2/RConn1
  Transform3/RConn1 -- F3/RConn1

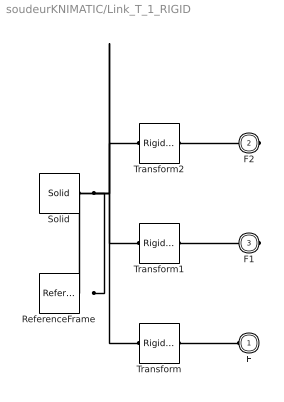
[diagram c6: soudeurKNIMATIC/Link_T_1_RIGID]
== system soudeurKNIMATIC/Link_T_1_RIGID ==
  ReferenceFrame : sm_lib/Frames and Transforms/Reference Frame
  Solid : sm_lib/Body Elements/Solid  InertiaType=Custom  Mass=smiData.Solid(1).mass  MassUnits=kg  CenterOfMass=smiData.Solid(1).CoM  CenterOfMassUnits=mm  MomentsOfInertia=smiData.Solid(1).MoI  MomentsOfInertiaUnits=kg*mm^2  ProductsOfInertia=smiData.Solid(1).PoI  ProductsOfInertiaUnits=kg*mm^2  DensityBased=on  Density=1000  DensityUnits=kg/m^3  DoExposeReferenceFrame=on  SerializedFrames=<Frames/>  GraphicType=FromGeometry  MarkerShape=Sphere  MarkerSize=10  GraphicVisPropType=SimpleVisualProperties  GraphicDiffuseColor=smiData.Solid(1).color  GraphicSpecularColor=[0.5 0.5 0.5 1.0]  GraphicAmbientColor=[0.15 0.15 0.15 1.0]  GraphicEmissiveColor=[0.0 0.0 0.0 1.0]  GraphicShininess=75  GraphicOpacity=smiData.Solid(1).opacity  GeometryShape=FromFile  RectangleSize=[1 1]  RectangleSizeUnits=m  BrickDimensions=[1 1 1]  BrickDimensionUnits=m  CylinderRadius=1  CylinderRadiusUnits=m  CylinderLength=1  CylinderLengthUnits=m  SphereRadius=1  SphereRadiusUnits=m  EllipsoidRadii=[1 1 1]  EllipsoidRadiiUnits=m  ExtrusionCrossSection=[1 1; -1 1; -1 -1; 1 -1]  ExtrusionCrossSectionUnits=m  ExtrusionLength=1  ExtrusionLengthUnits=m  PolygonNumSides=3  PolygonOuterRadius=1  PolygonOuterRadiusUnits=m  ExtGeomFileType=STEP  ExtGeomFileName=Link_T_Default_sldprt.STEP  ExtGeomFileUnits=m  RevolutionCrossSection=[1 1; 1 -1; 2 -1; 2 1]  RevolutionCrossSectionUnits=m  RevolutionExtent=Full  RevolutionAngle=180  RevolutionAngleUnits=deg
  Transform : sm_lib/Frames and Transforms/Rigid Transform  TranslationMethod=Cartesian  TranslationStandardOffset=0  TranslationLengthUnit=mm  TranslationStandardAxis=+Z  TranslationCartesianOffset=smiData.RigidTransform(2).translation  TranslationROffset=0  TranslationROffsetUnits=m  TranslationZOffset=0  TranslationZOffsetUnits=m  TranslationThetaOffset=0  TranslationThetaOffsetUnits=deg  RotationMethod=ArbitraryAxis  RotationAngleUnits=rad  RotationStandardAxis=+Z  RotationAngle=smiData.RigidTransform(2).angle  RotationArbitraryAxis=smiData.RigidTransform(2).axis  FollAlignAxisA=+X  BaseAlignAxisA=+Y  FollAlignAxisB=+Y  BaseAlignAxisB=+Z  RotationSequenceAxes=FollowerAxes  RotationSequence=XYX  RotationSequenceAngles=[0 0 0]  RotationSequenceAnglesUnits=deg  RotationMatrix=[1 0 0; 0 1 0; 0 0 1]
  Transform1 : sm_lib/Frames and Transforms/Rigid Transform  TranslationMethod=Cartesian  TranslationStandardOffset=0  TranslationLengthUnit=mm  TranslationStandardAxis=+Z  TranslationCartesianOffset=smiData.RigidTransform(3).translation  TranslationROffset=0  TranslationROffsetUnits=m  TranslationZOffset=0  TranslationZOffsetUnits=m  TranslationThetaOffset=0  TranslationThetaOffsetUnits=deg  RotationMethod=ArbitraryAxis  RotationAngleUnits=rad  RotationStandardAxis=+Z  RotationAngle=smiData.RigidTransform(3).angle  RotationArbitraryAxis=smiData.RigidTransform(3).axis  FollAlignAxisA=+X  BaseAlignAxisA=+Y  FollAlignAxisB=+Y  BaseAlignAxisB=+Z  RotationSequenceAxes=FollowerAxes  RotationSequence=XYX  RotationSequenceAngles=[0 0 0]  RotationSequenceAnglesUnits=deg  RotationMatrix=[1 0 0; 0 1 0; 0 0 1]
  Transform2 : sm_lib/Frames and Transforms/Rigid Transform  TranslationMethod=Cartesian  TranslationStandardOffset=0  TranslationLengthUnit=mm  TranslationStandardAxis=+Z  TranslationCartesianOffset=smiData.RigidTransform(5).translation  TranslationROffset=0  TranslationROffsetUnits=m  TranslationZOffset=0  TranslationZOffsetUnits=m  TranslationThetaOffset=0  TranslationThetaOffsetUnits=deg  RotationMethod=ArbitraryAxis  RotationAngleUnits=rad  RotationStandardAxis=+Z  RotationAngle=smiData.RigidTransform(5).angle  RotationArbitraryAxis=smiData.RigidTransform(5).axis  FollAlignAxisA=+X  BaseAlignAxisA=+Y  FollAlignAxisB=+Y  BaseAlignAxisB=+Z  RotationSequenceAxes=FollowerAxes  RotationSequence=XYX  RotationSequenceAngles=[0 0 0]  RotationSequenceAnglesUnits=deg  RotationMatrix=[1 0 0; 0 1 0; 0 0 1]
  F : PMIOPort  Side=Left
  F2 : PMIOPort  Port=2  Side=Right
  F1 : PMIOPort  Port=3  Side=Right
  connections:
  Solid/RConn1 -- ReferenceFrame/RConn1 -- Transform/LConn1 -- Transform1/LConn1 -- Transform2/LConn1
  Transform/RConn1 -- F/RConn1
  Transform1/RConn1 -- F1/RConn1
  Transform2/RConn1 -- F2/RConn1

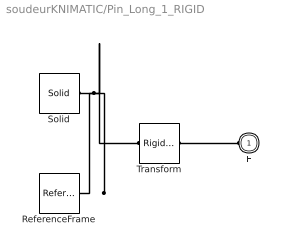
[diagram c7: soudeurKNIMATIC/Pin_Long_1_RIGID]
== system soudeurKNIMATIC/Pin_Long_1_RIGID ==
  ReferenceFrame : sm_lib/Frames and Transforms/Reference Frame
  Solid : sm_lib/Body Elements/Solid  InertiaType=Custom  Mass=smiData.Solid(7).mass  MassUnits=kg  CenterOfMass=smiData.Solid(7).CoM  CenterOfMassUnits=mm  MomentsOfInertia=smiData.Solid(7).MoI  MomentsOfInertiaUnits=kg*mm^2  ProductsOfInertia=smiData.Solid(7).PoI  ProductsOfInertiaUnits=kg*mm^2  DensityBased=on  Density=1000  DensityUnits=kg/m^3  DoExposeReferenceFrame=on  SerializedFrames=<Frames/>  GraphicType=FromGeometry  MarkerShape=Sphere  MarkerSize=10  GraphicVisPropType=SimpleVisualProperties  GraphicDiffuseColor=smiData.Solid(7).color  GraphicSpecularColor=[0.5 0.5 0.5 1.0]  GraphicAmbientColor=[0.15 0.15 0.15 1.0]  GraphicEmissiveColor=[0.0 0.0 0.0 1.0]  GraphicShininess=75  GraphicOpacity=smiData.Solid(7).opacity  GeometryShape=FromFile  RectangleSize=[1 1]  RectangleSizeUnits=m  BrickDimensions=[1 1 1]  BrickDimensionUnits=m  CylinderRadius=1  CylinderRadiusUnits=m  CylinderLength=1  CylinderLengthUnits=m  SphereRadius=1  SphereRadiusUnits=m  EllipsoidRadii=[1 1 1]  EllipsoidRadiiUnits=m  ExtrusionCrossSection=[1 1; -1 1; -1 -1; 1 -1]  ExtrusionCrossSectionUnits=m  ExtrusionLength=1  ExtrusionLengthUnits=m  PolygonNumSides=3  PolygonOuterRadius=1  PolygonOuterRadiusUnits=m  ExtGeomFileType=STEP  ExtGeomFileName=Pin_Long_Default_sldprt.STEP  ExtGeomFileUnits=m  RevolutionCrossSection=[1 1; 1 -1; 2 -1; 2 1]  RevolutionCrossSectionUnits=m  RevolutionExtent=Full  RevolutionAngle=180  RevolutionAngleUnits=deg
  Transform : sm_lib/Frames and Transforms/Rigid Transform  TranslationMethod=Cartesian  TranslationStandardOffset=0  TranslationLengthUnit=mm  TranslationStandardAxis=+Z  TranslationCartesianOffset=smiData.RigidTransform(6).translation  TranslationROffset=0  TranslationROffsetUnits=m  TranslationZOffset=0  TranslationZOffsetUnits=m  TranslationThetaOffset=0  TranslationThetaOffsetUnits=deg  RotationMethod=ArbitraryAxis  RotationAngleUnits=rad  RotationStandardAxis=+Z  RotationAngle=smiData.RigidTransform(6).angle  RotationArbitraryAxis=smiData.RigidTransform(6).axis  FollAlignAxisA=+X  BaseAlignAxisA=+Y  FollAlignAxisB=+Y  BaseAlignAxisB=+Z  RotationSequenceAxes=FollowerAxes  RotationSequence=XYX  RotationSequenceAngles=[0 0 0]  RotationSequenceAnglesUnits=deg  RotationMatrix=[1 0 0; 0 1 0; 0 0 1]
  F : PMIOPort  Side=Left
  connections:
  Solid/RConn1 -- ReferenceFrame/RConn1 -- Transform/LConn1
  Transform/RConn1 -- F/RConn1

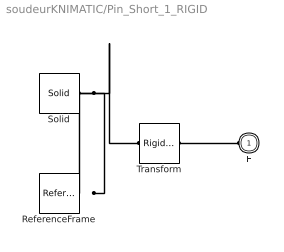
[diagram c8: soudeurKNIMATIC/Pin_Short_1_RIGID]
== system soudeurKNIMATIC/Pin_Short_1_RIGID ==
  ReferenceFrame : sm_lib/Frames and Transforms/Reference Frame
  Solid : sm_lib/Body Elements/Solid  InertiaType=Custom  Mass=smiData.Solid(3).mass  MassUnits=kg  CenterOfMass=smiData.Solid(3).CoM  CenterOfMassUnits=mm  MomentsOfInertia=smiData.Solid(3).MoI  MomentsOfInertiaUnits=kg*mm^2  ProductsOfInertia=smiData.Solid(3).PoI  ProductsOfInertiaUnits=kg*mm^2  DensityBased=on  Density=1000  DensityUnits=kg/m^3  DoExposeReferenceFrame=on  SerializedFrames=<Frames/>  GraphicType=FromGeometry  MarkerShape=Sphere  MarkerSize=10  GraphicVisPropType=SimpleVisualProperties  GraphicDiffuseColor=smiData.Solid(3).color  GraphicSpecularColor=[0.5 0.5 0.5 1.0]  GraphicAmbientColor=[0.15 0.15 0.15 1.0]  GraphicEmissiveColor=[0.0 0.0 0.0 1.0]  GraphicShininess=75  GraphicOpacity=smiData.Solid(3).opacity  GeometryShape=FromFile  RectangleSize=[1 1]  RectangleSizeUnits=m  BrickDimensions=[1 1 1]  BrickDimensionUnits=m  CylinderRadius=1  CylinderRadiusUnits=m  CylinderLength=1  CylinderLengthUnits=m  SphereRadius=1  SphereRadiusUnits=m  EllipsoidRadii=[1 1 1]  EllipsoidRadiiUnits=m  ExtrusionCrossSection=[1 1; -1 1; -1 -1; 1 -1]  ExtrusionCrossSectionUnits=m  ExtrusionLength=1  ExtrusionLengthUnits=m  PolygonNumSides=3  PolygonOuterRadius=1  PolygonOuterRadiusUnits=m  ExtGeomFileType=STEP  ExtGeomFileName=Pin_Short_Default_sldprt.STEP  ExtGeomFileUnits=m  RevolutionCrossSection=[1 1; 1 -1; 2 -1; 2 1]  RevolutionCrossSectionUnits=m  RevolutionExtent=Full  RevolutionAngle=180  RevolutionAngleUnits=deg
  Transform : sm_lib/Frames and Transforms/Rigid Transform  TranslationMethod=Cartesian  TranslationStandardOffset=0  TranslationLengthUnit=mm  TranslationStandardAxis=+Z  TranslationCartesianOffset=smiData.RigidTransform(18).translation  TranslationROffset=0  TranslationROffsetUnits=m  TranslationZOffset=0  TranslationZOffsetUnits=m  TranslationThetaOffset=0  TranslationThetaOffsetUnits=deg  RotationMethod=ArbitraryAxis  RotationAngleUnits=rad  RotationStandardAxis=+Z  RotationAngle=smiData.RigidTransform(18).angle  RotationArbitraryAxis=smiData.RigidTransform(18).axis  FollAlignAxisA=+X  BaseAlignAxisA=+Y  FollAlignAxisB=+Y  BaseAlignAxisB=+Z  RotationSequenceAxes=FollowerAxes  RotationSequence=XYX  RotationSequenceAngles=[0 0 0]  RotationSequenceAnglesUnits=deg  RotationMatrix=[1 0 0; 0 1 0; 0 0 1]
  F : PMIOPort  Side=Left
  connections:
  Solid/RConn1 -- ReferenceFrame/RConn1 -- Transform/LConn1
  Transform/RConn1 -- F/RConn1

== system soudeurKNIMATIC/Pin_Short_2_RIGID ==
  ReferenceFrame : sm_lib/Frames and Transforms/Reference Frame
  Solid : sm_lib/Body Elements/Solid  InertiaType=Custom  Mass=smiData.Solid(3).mass  MassUnits=kg  CenterOfMass=smiData.Solid(3).CoM  CenterOfMassUnits=mm  MomentsOfInertia=smiData.Solid(3).MoI  MomentsOfInertiaUnits=kg*mm^2  ProductsOfInertia=smiData.Solid(3).PoI  ProductsOfInertiaUnits=kg*mm^2  DensityBased=on  Density=1000  DensityUnits=kg/m^3  DoExposeReferenceFrame=on  SerializedFrames=<Frames/>  GraphicType=FromGeometry  MarkerShape=Sphere  MarkerSize=10  GraphicVisPropType=SimpleVisualProperties  GraphicDiffuseColor=smiData.Solid(3).color  GraphicSpecularColor=[0.5 0.5 0.5 1.0]  GraphicAmbientColor=[0.15 0.15 0.15 1.0]  GraphicEmissiveColor=[0.0 0.0 0.0 1.0]  GraphicShininess=75  GraphicOpacity=smiData.Solid(3).opacity  GeometryShape=FromFile  RectangleSize=[1 1]  RectangleSizeUnits=m  BrickDimensions=[1 1 1]  BrickDimensionUnits=m  CylinderRadius=1  CylinderRadiusUnits=m  CylinderLength=1  CylinderLengthUnits=m  SphereRadius=1  SphereRadiusUnits=m  EllipsoidRadii=[1 1 1]  EllipsoidRadiiUnits=m  ExtrusionCrossSection=[1 1; -1 1; -1 -1; 1 -1]  ExtrusionCrossSectionUnits=m  ExtrusionLength=1  ExtrusionLengthUnits=m  PolygonNumSides=3  PolygonOuterRadius=1  PolygonOuterRadiusUnits=m  ExtGeomFileType=STEP  ExtGeomFileName=Pin_Short_Default_sldprt.STEP  ExtGeomFileUnits=m  RevolutionCrossSection=[1 1; 1 -1; 2 -1; 2 1]  RevolutionCrossSectionUnits=m  RevolutionExtent=Full  RevolutionAngle=180  RevolutionAngleUnits=deg
  Transform : sm_lib/Frames and Transforms/Rigid Transform  TranslationMethod=Cartesian  TranslationStandardOffset=0  TranslationLengthUnit=mm  TranslationStandardAxis=+Z  TranslationCartesianOffset=smiData.RigidTransform(20).translation  TranslationROffset=0  TranslationROffsetUnits=m  TranslationZOffset=0  TranslationZOffsetUnits=m  TranslationThetaOffset=0  TranslationThetaOffsetUnits=deg  RotationMethod=ArbitraryAxis  RotationAngleUnits=rad  RotationStandardAxis=+Z  RotationAngle=smiData.RigidTransform(20).angle  RotationArbitraryAxis=smiData.RigidTransform(20).axis  FollAlignAxisA=+X  BaseAlignAxisA=+Y  FollAlignAxisB=+Y  BaseAlignAxisB=+Z  RotationSequenceAxes=FollowerAxes  RotationSequence=XYX  RotationSequenceAngles=[0 0 0]  RotationSequenceAnglesUnits=deg  RotationMatrix=[1 0 0; 0 1 0; 0 0 1]
  F : PMIOPort  Side=Left
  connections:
  Solid/RConn1 -- ReferenceFrame/RConn1 -- Transform/LConn1
  Transform/RConn1 -- F/RConn1

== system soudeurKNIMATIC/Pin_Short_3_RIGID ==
  ReferenceFrame : sm_lib/Frames and Transforms/Reference Frame
  Solid : sm_lib/Body Elements/Solid  InertiaType=Custom  Mass=smiData.Solid(3).mass  MassUnits=kg  CenterOfMass=smiData.Solid(3).CoM  CenterOfMassUnits=mm  MomentsOfInertia=smiData.Solid(3).MoI  MomentsOfInertiaUnits=kg*mm^2  ProductsOfInertia=smiData.Solid(3).PoI  ProductsOfInertiaUnits=kg*mm^2  DensityBased=on  Density=1000  DensityUnits=kg/m^3  DoExposeReferenceFrame=on  SerializedFrames=<Frames/>  GraphicType=FromGeometry  MarkerShape=Sphere  MarkerSize=10  GraphicVisPropType=SimpleVisualProperties  GraphicDiffuseColor=smiData.Solid(3).color  GraphicSpecularColor=[0.5 0.5 0.5 1.0]  GraphicAmbientColor=[0.15 0.15 0.15 1.0]  GraphicEmissiveColor=[0.0 0.0 0.0 1.0]  GraphicShininess=75  GraphicOpacity=smiData.Solid(3).opacity  GeometryShape=FromFile  RectangleSize=[1 1]  RectangleSizeUnits=m  BrickDimensions=[1 1 1]  BrickDimensionUnits=m  CylinderRadius=1  CylinderRadiusUnits=m  CylinderLength=1  CylinderLengthUnits=m  SphereRadius=1  SphereRadiusUnits=m  EllipsoidRadii=[1 1 1]  EllipsoidRadiiUnits=m  ExtrusionCrossSection=[1 1; -1 1; -1 -1; 1 -1]  ExtrusionCrossSectionUnits=m  ExtrusionLength=1  ExtrusionLengthUnits=m  PolygonNumSides=3  PolygonOuterRadius=1  PolygonOuterRadiusUnits=m  ExtGeomFileType=STEP  ExtGeomFileName=Pin_Short_Default_sldprt.STEP  ExtGeomFileUnits=m  RevolutionCrossSection=[1 1; 1 -1; 2 -1; 2 1]  RevolutionCrossSectionUnits=m  RevolutionExtent=Full  RevolutionAngle=180  RevolutionAngleUnits=deg
  Transform : sm_lib/Frames and Transforms/Rigid Transform  TranslationMethod=Cartesian  TranslationStandardOffset=0  TranslationLengthUnit=mm  TranslationStandardAxis=+Z  TranslationCartesianOffset=smiData.RigidTransform(21).translation  TranslationROffset=0  TranslationROffsetUnits=m  TranslationZOffset=0  TranslationZOffsetUnits=m  TranslationThetaOffset=0  TranslationThetaOffsetUnits=deg  RotationMethod=ArbitraryAxis  RotationAngleUnits=rad  RotationStandardAxis=+Z  RotationAngle=smiData.RigidTransform(21).angle  RotationArbitraryAxis=smiData.RigidTransform(21).axis  FollAlignAxisA=+X  BaseAlignAxisA=+Y  FollAlignAxisB=+Y  BaseAlignAxisB=+Z  RotationSequenceAxes=FollowerAxes  RotationSequence=XYX  RotationSequenceAngles=[0 0 0]  RotationSequenceAnglesUnits=deg  RotationMatrix=[1 0 0; 0 1 0; 0 0 1]
  F : PMIOPort  Side=Right
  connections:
  Solid/RConn1 -- ReferenceFrame/RConn1 -- Transform/LConn1
  Transform/RConn1 -- F/RConn1
